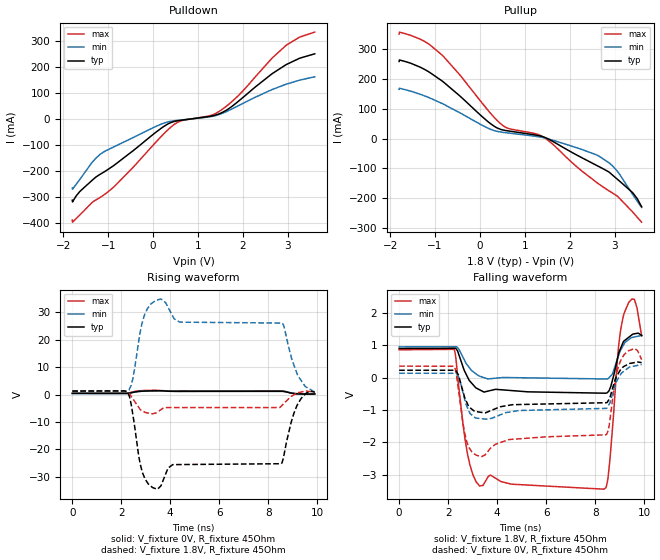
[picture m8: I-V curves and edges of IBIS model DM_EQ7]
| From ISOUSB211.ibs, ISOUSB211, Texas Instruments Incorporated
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[Model]   DM_EQ7
Model_type   Output
Polarity   Inverting
Vmeas = 0.2
Vref = 0
Cref = 15pF
Rref = 45
|   typ   min   max
C_comp   5pF   3pF   8pF
[Voltage Range]   1.8   1.71   1.89
[Temperature Range]   27   150   -40
[Pullup Reference]   1.8   1.71   1.89
[Pulldown Reference]   0   0   0
[Power Clamp Reference]   1.8   1.71   1.89
[GND Clamp Reference]   0   0   0
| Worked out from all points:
|   slope of the pulldown table from 0 to 0.27 V, typ, clamps not added: 7.95 ohm
|   slope of the pullup table from 0 to 0.27 V, typ, clamps not added: 7.94 ohm
|   falling waveform, V_fixture 1.8V, R_fixture 45Ohm: 20-80 % time 252ps typ, 310ps min, 40.9ps max; typ from 0.895 V to 1.3 V
|   rising waveform, V_fixture 0V, R_fixture 45Ohm: 20-80 % time 184ps typ, 235ps min, 124ps max; typ from 0.46 V to 0.225 V
|   rising waveform, V_fixture 1.8V, R_fixture 45Ohm: 20-80 % time 71.7ps typ, 40.9ps min, 34.1ps max; typ from 1.3 V to 0.895 V
|   falling waveform, V_fixture 0V, R_fixture 45Ohm: 20-80 % time 286ps typ, 394ps min, 61.1ps max; typ from 0.225 V to 0.46 V
[Pulldown]
|   Voltage   I(typ)   I(min)   I(max)
-1.8V     -312.3mA   -266.2mA   -388.8mA
-1.795V   -319mA     -269.8mA   -396.8mA
-1.633V   -278.9mA   -232.8mA   -369.2mA
-1.179V   -212.7mA   -136mA     -301.6mA
-865.8mV  -177.8mA   -106.8mA   -260mA
73.8mV    -49.63mA   -27.98mA   -87.09mA
538.2mV   -7.266mA   -5.626mA   -13.71mA
1.294V    10.85mA    9.019mA    13.98mA
1.521V    23.18mA    20.15mA    34.45mA
1.899V    67.71mA    50.57mA    89.7mA
2.947V    206.8mA    132.3mA    280.4mA
3.6V      250.2mA    161.9mA    333.6mA
[Pullup]
|   Voltage   I(typ)   I(min)   I(max)
-1.8V     259.8mA    166.3mA    352.1mA
-1.795V   264.8mA    169.7mA    358.5mA
-1.325V   240.1mA    149.1mA    334.3mA
-849.6mV  194.9mA    118.9mA    282mA
381.6mV   36.3mA     24.84mA    61.51mA
613.8mV   26.64mA    19.55mA    35.63mA
1.402V    6.733mA    3.773mA    6.537mA
2.612V    -90.76mA   -55.24mA   -148.5mA
2.876V    -112.3mA   -81.28mA   -175.5mA
3.065V    -136.9mA   -110.7mA   -193.6mA
3.4V      -181.3mA   -187.3mA   -246.2mA
3.6V      -228.6mA   -231.2mA   -280.5mA
[Ramp]
R_load = 45
|   typ   min   max
dV/dt_r   0.140808/1.94051e-10   0.160407/1.92207e-10   0.120509/1.27944e-10
dV/dt_f   0.243789/2.10846e-10   0.210518/3.18986e-10   0.256824/3.78667e-11
[Falling Waveform]
V_fixture = 1.8V
V_fixture_min = 1.71V
V_fixture_max = 1.89V
R_fixture = 45Ohm
C_fixture = 0F
|   Time   V(typ)   V(min)   V(max)
0s        895mV      947.6mV    856.5mV
2.245ns   904.1mV    951.5mV    871.2mV
2.776ns   39.82mV    393mV      -2.301V
3.277ns   -375.8mV   44.21mV    -3.343V
8.356ns   -483mV     -43.7mV    -3.446V
8.523ns   -448.5mV   -38.95mV   -3.13V
8.96ns    738.7mV    683.2mV    972.2mV
9.15ns    1.097V     991mV      1.886V
9.59ns    1.349V     1.249V     2.419V
9.9ns     1.301V     1.298V     1.285V
[Rising Waveform]
V_fixture = 0V
V_fixture_min = 0V
V_fixture_max = 0V
R_fixture = 45Ohm
C_fixture = 0F
|   Time   V(typ)   V(min)   V(max)
0s        459.5mV    400.3mV    553.4mV
2.213ns   455mV      400.3mV    551.8mV
2.719ns   1.173V     1.127V     1.393V
3.39ns    1.384V     1.388V     1.593V
3.723ns   1.364V     1.421V     1.425V
4.393ns   1.197V     1.176V     1.377V
8.608ns   1.19V      1.219V     1.278V
8.914ns   615.5mV    676mV      601.3mV
9.086ns   379.7mV    345.1mV    403.3mV
9.9ns     224.9mV    133mV      352.5mV
[Rising Waveform]
V_fixture = 1.8V
V_fixture_min = 1.71V
V_fixture_max = 1.89V
R_fixture = 45Ohm
C_fixture = 0F
|   Time   V(typ)   V(min)   V(max)
0s        1.301V     1.298V     1.285V
2.257ns   941.5mV    1.533V     797.7mV
2.476ns   -7.456V    5.958V     -1.549V
2.855ns   -28.12V    26.21V     -5.898V
3.46ns    -34.49V    34.49V     -6.474V
3.806ns   -29.11V    33.63V     -4.816V
4.105ns   -25.53V    28.56V     -4.712V
8.533ns   -25.21V    26.11V     -4.178V
9.166ns   -4.157V    7.919V     606mV
9.9ns     895mV      947.6mV    856.5mV
[Falling Waveform]
|Gnd
V_fixture = 0V
V_fixture_min = 0V
V_fixture_max = 0V
R_fixture = 45Ohm
C_fixture = 0F
|   Time   V(typ)   V(min)   V(max)
0s        224.9mV    133mV      352.5mV
2.245ns   224.9mV    131mV      347.5mV
2.761ns   -763.2mV   -877.5mV   -1.981V
3.359ns   -1.076V    -1.27V     -2.437V
4.462ns   -859.7mV   -1.071V    -1.92V
8.444ns   -777.3mV   -952.2mV   -1.769V
8.85ns    -7.652mV   -176.6mV   29.44mV
9.059ns   264.6mV    118.3mV    547.4mV
9.607ns   460.8mV    355mV      893.1mV
9.9ns     459.5mV    400.3mV    553.4mV
